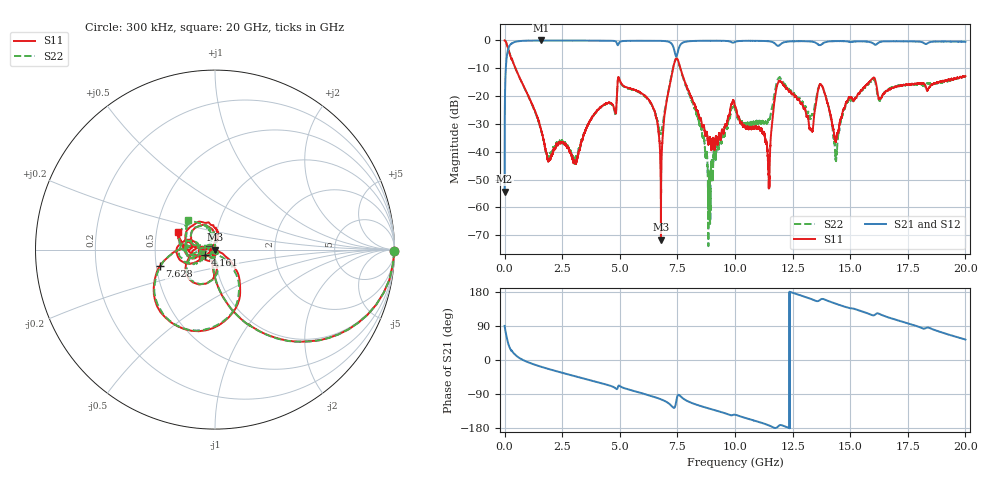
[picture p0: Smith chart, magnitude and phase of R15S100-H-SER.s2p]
!{R15S100}
!Johanson Technology Inc.
!www.johansontechnology.com
!Test Board Conditions:
!Substrate Type  RO4350B
!Substrate Thickness  20 mil
!Substrate Dk  3.66
!TL Type: GCPW
!TL Trace Width  34 mil
!TL Gap  10 mil
!Electrode orientation  Horizontal
!DUT TOPOLOGY	SERIES
!Mounting Pad LxW  26x52 mil
! Created Sat Feb  6 14:04:39 2021
# hz S ma R 50
! 2 Port Network Data from SP1.SP block
! freq  magS11  angS11  magS21  angS21  magS12  angS12  magS22  angS22
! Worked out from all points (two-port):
!   20001 points, 300 kHz to 20 GHz, reference 50 ohm
!   highest |S21| = -0.02 dB at 1.575 GHz (marker M1); lowest = -54.3 dB at 300 kHz (marker M2)
!   |S21| within 3 dB of the highest: 159.7 MHz to 7.35 GHz (7.19 GHz wide, 191 % of centre); 7.553 GHz to end of sweep
!   lowest |S11| = -71.5 dB at 6.785 GHz (marker M3), VSWR 1.00, Z = 50 - j0.0259 ohm
!   |S11| at or under -10 dB: 470.8 MHz to 7.31 GHz (6.839 GHz wide, 176 % of centre); 7.632 GHz to end of sweep
!   |S22| runs from -73.9 to 0.0 dB; largest |S21 - S12| = 0.016
!   S11 on the Smith chart (normalised r, x): 300 kHz: open; 4.161 GHz: 0.89, -0.06; 7.628 GHz: 0.52, -0.11; 20 GHz: 0.65, +0.14
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300000  1 -0.4  0.00193 90.0  0.001946 89.3  0.9992 -0.3
1.043e8  0.8338 -34.5  0.5474 55.3  0.5486 55.2  0.8342 -34.5
2.003e8  0.6143 -54.1  0.783 35.5  0.7835 35.4  0.6152 -54.2
1.5753e9  0.02546 -119.1  0.9983 -17.6  0.9963 -17.6  0.02486 -93.4
1.9313e9  0.007122 163.4  0.9969 -24.1  0.9969 -24.1  0.006951 -24.4
3.3343e9  0.01541 -155.4  0.9949 -47.3  0.9937 -47.3  0.01636 -116.8
4.1613e9  0.06302 -150.3  0.9904 -60.7  0.9893 -60.7  0.06214 -150.9
5.0043e9  0.19 -149.5  0.9443 -68.9  0.944 -68.9  0.1855 -148.2
6.6673e9  0.02505 159.6  0.986 -101.0  0.9867 -101.0  0.03158 -151.4
6.7853e9  0.0002647 -78.4  0.9844 -103.7  0.9837 -103.7  0.02201 -101.8
7.3103e9  0.3165 -65.2  0.7895 -125.2  0.7892 -125.1  0.3207 -67.5
7.6283e9  0.3199 -163.6  0.8342 -95.2  0.8359 -95.2  0.31 -164.5
8.9003e9  0.01793 -158.5  0.9872 -128.6  0.9874 -128.5  0.00354 114.8
1.00003e10  0.06583 177.3  0.9398 -144.2  0.9408 -144.2  0.05652 172.8
1.14363e10  0.006472 120.9  0.9689 -171.8  0.9701 -171.8  0.03669 166.1
1.19273e10  0.1892 144.3  0.8198 -172.6  0.8196 -172.6  0.217 149.3
1.33343e10  0.02377 144.1  0.9531 160.3  0.9537 160.2  0.04552 146.9
1.37363e10  0.1611 128.0  0.8382 160.5  0.8372 160.3  0.1636 130.6
1.43793e10  0.01588 148.5  0.975 148.3  0.9726 148.2  0.007366 169.0
1.49093e10  0.08734 -151.5  0.9557 137.9  0.9557 137.8  0.08012 -143.5
1.66673e10  0.1322 -159.4  0.9687 112.0  0.9594 111.9  0.1332 -159.2
2e10  0.2289 153.8  0.946 53.9  0.9398 53.5  0.2248 132.4
